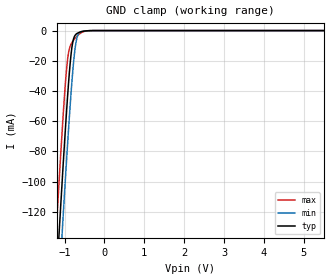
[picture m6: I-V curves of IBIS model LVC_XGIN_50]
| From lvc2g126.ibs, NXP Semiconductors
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|   Model LVC_XGIN_50
[Model]   LVC_XGIN_50
Model_type   Input
Vinl =   1.5V
Vinh =   3.5V
C_comp   2.89pF   1.97pF   3.94pF
[Model Spec]
| Note: The input and output voltage ratings may be exceeded if the input and
|   output current ratings are observed (please refer to the data sheet)
|   Subparameter   typ   min   max
| Thresholds
Vinh   3.5   3.15   3.85
Vinl   1.5   1.35   1.65
| Overshoot
S_overshoot_high   6.5   6.5   6.5   | Static overshoot
S_overshoot_low   -0.5   -0.5   -0.5
D_overshoot_high   11.0   11.0   11.0   | Dynamic overshoot
D_overshoot_low   -0.95   -0.9   -1.0
D_overshoot_time   3n   3n   3n
|Ambient temperature:   25   85   -40
[Temperature Range]   50   105   -10
[Voltage Range]   5.0V   4.5V   5.5V
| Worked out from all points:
|   GND clamp passes 1 mA (typ) near -0.61 V on its own axis
|Process Range   nominal   slow   fast
[GND_clamp]
| voltage   I(typ)   I(min)   I(max)
-5.5V     -2.277A    -2.307A    -2.246A
-1.221V   -173.6mA   -208.2mA   -138.8mA
-1.2V     -163.7mA   -198.3mA   -129mA
-1.136V   -134.3mA   -168.7mA   -99.82mA
-1.071V   -105.4mA   -139.6mA   -71.73mA
-1.05V    -95.98mA   -130mA     -62.73mA
-942.9mV  -51.21mA   -83.48mA   -24.05mA
-900mV    -35.22mA   -65.87mA   -14.8mA
-835.7mV  -15.71mA   -41.31mA   -9.021mA
-728.6mV  -2.901mA   -10.64mA   -4.899mA
-642.9mV  -1.321mA   -1.88mA    -2.576mA
5.5V      0A         0A         0A
